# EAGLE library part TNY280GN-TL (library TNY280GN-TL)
AC/DC Converters 28.5W 85-265 VAC 36.5W/230 VAC Source: Datasheet
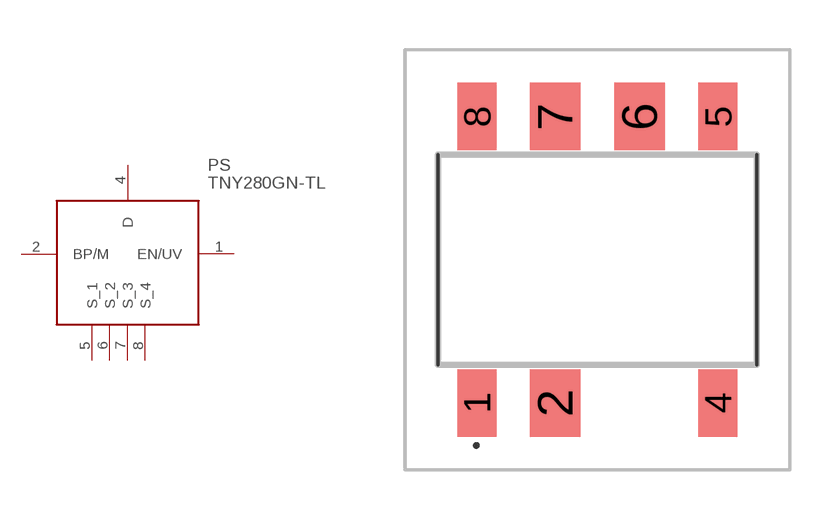
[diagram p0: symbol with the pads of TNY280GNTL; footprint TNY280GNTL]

Designator prefix PS

## TNY280GN-TL (Description: AC/DC Converters 28.5W 85-265 VAC 36.5W/230 VAC; Height: 3.98mm; Manufacturer_Name: Power Integrations; Manufacturer_Part_Number: TNY280GN-TL; Mouser_Part_Number: 869-TNY280GN-TL; Mouser_Price-Stock: https://www.mouser.co.uk/ProductDetail/Power-Integrations/TNY280GN-TL?qs=vF78I%252BjhbY8Q8Coo9C8agA%3D%3D)  [TNY280GNTL]
1  EN/UV
2  BP/M
4  D
5  S_1
6  S_2
7  S_3
8  S_4

## Footprint TNY280GNTL (pad centres in mm)
SMD-8C_1
smd 1.168 x 2.032: 1 -3.632,-4.318; 4 3.632,-4.318; 5 3.632,4.318; 8 -3.632,4.318
smd 1.524 x 2.032: 2 -1.27,-4.318; 6 1.27,4.318; 7 -1.27,4.318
